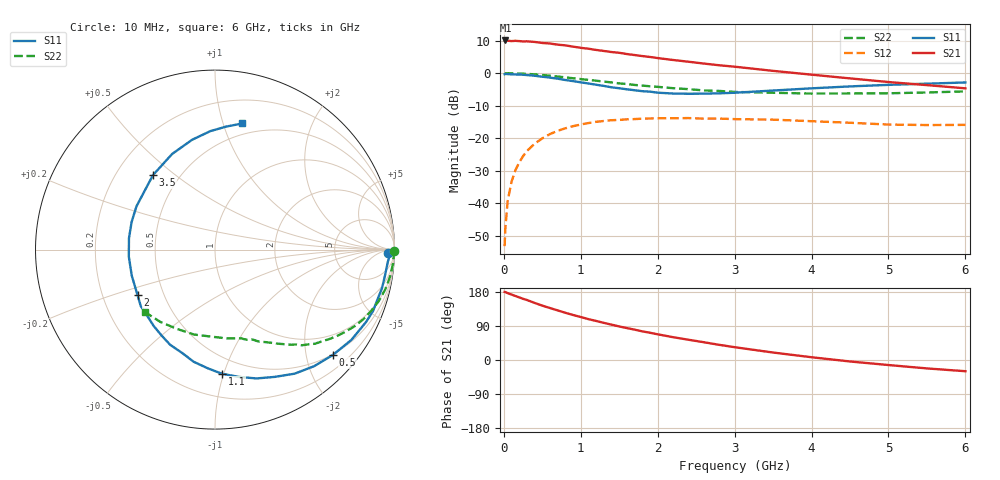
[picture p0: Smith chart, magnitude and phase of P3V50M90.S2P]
! SIEMENS Small Signal Semiconductors
! BFP181
! Si NPN RF Bipolar Junction Transistor in SOT143
! VCE = 0.5 V  IC = 0.9 mA
! Common Emitter S-Parameters:  March  1996
# GHz  S  MA  R  50
!  f  S11  S21  S12  S22
! GHz  MAG  ANG  MAG  ANG  MAG  ANG  MAG  ANG
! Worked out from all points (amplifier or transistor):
!   36 points, 10 MHz to 6 GHz, reference 50 ohm
!   highest |S21| = 10.0 dB at 20 MHz (marker M1)
!   |S21| within 3 dB of that: start of sweep to 1.229 GHz
!   unconditionally stable (mu >= 1): 2.771 GHz to end of sweep
!   at 250 MHz: K = 0.10, MSG = 17.6 dB, |S12| = -25.5 dB
!   at 1.4 GHz: K = 0.55, MSG = 10.5 dB, |S12| = -14.5 dB
!   at 6 GHz: K = 1.56, MAG = 1.2 dB, |S12| = -15.9 dB
!   S11 on the Smith chart (normalised r, x): 10 MHz: 42, -19; 500 MHz: 0.48, -2.54; 1.1 GHz: 0.37, -0.99; 2 GHz: 0.35, -0.24; 3.5 GHz: 0.36, +0.42; 6 GHz: 0.40, +1.16
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0.01  0.9614 -1.0  3.118 179.6  0.0022 90.4  0.9982 -0.5
0.02  0.9735 -1.9  3.174 179.2  0.0042 87.3  0.9913 -0.8
0.05  0.9652 -4.1  3.15 176.4  0.011 89.1  0.996 -2.3
0.1  0.9581 -8.7  3.102 172.7  0.0215 84.5  0.9948 -4.4
0.15  0.955 -12.9  3.135 168.9  0.0322 80.8  0.9902 -6.7
0.3  0.9331 -25.7  3.078 158.4  0.0636 72.8  0.9735 -13.3
0.4  0.9114 -33.5  3.011 150.6  0.0823 67.4  0.9563 -17.5
0.5  0.8809 -41.8  2.904 143.5  0.0996 61.9  0.9351 -21.4
0.6  0.8527 -49.6  2.848 137.1  0.1159 56.7  0.9128 -25.2
0.8  0.7832 -64.9  2.669 124.6  0.1421 47.6  0.8602 -32.0
1.1  0.693 -86.7  2.37 107.8  0.1711 35.4  0.7863 -40.5
1.3  0.636 -100.8  2.189 98.0  0.1841 28.4  0.7415 -45.4
1.5  0.586 -115.3  2.051 88.5  0.191 22.7  0.6948 -49.5
1.8  0.5278 -135.8  1.827 75.6  0.1996 15.5  0.6445 -54.7
2  0.5007 -149.5  1.703 67.8  0.2028 11.3  0.6155 -57.8
2.2  0.4859 -162.6  1.591 60.2  0.2028 7.0  0.5871 -61.4
2.8  0.4894 161.7  1.32 40.0  0.2005 -2.4  0.5328 -70.6
3.5  0.5401 129.8  1.083 19.7  0.1929 -9.9  0.4993 -82.3
4  0.5841 114.1  0.947 7.3  0.1826 -14.1  0.4852 -92.7
4.5  0.6249 101.8  0.83 -3.9  0.1729 -17.7  0.4874 -104.0
5.5  0.6886 84.7  0.654 -22.2  0.1594 -16.3  0.5047 -126.9
6  0.7189 77.8  0.584 -29.6  0.1604 -15.3  0.5237 -138.4
